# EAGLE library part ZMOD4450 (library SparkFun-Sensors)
ZMOD4450 Food-Ripening Gas Sensor The ZMOD4450 gas sensor module is a software configurable platform designed for detecting gases associated with food ripening or rotting and is targeted for use in refrigeration air quality (RAQ) applications. The sensor is a 12-pin LGA assembly (3.0 x 3.0 x 0.7 mm) that consists of a gas sense element and a CMOS signal conditioning IC. The module’s sense element consists of a micro-heater and sensing material integrated on a silicon-based MEMS structure. It measures the metal oxide (MOx) conductivity, which is a function of the gas concentration. SparkFun Products: SparkFun Refrigeration Gas Sensor ZMOD4450 (Qwiic)
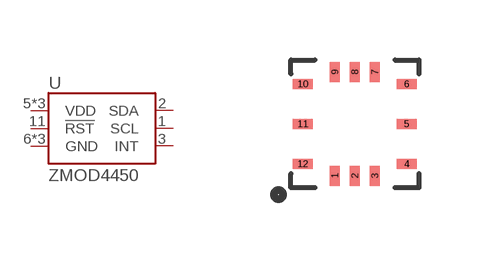
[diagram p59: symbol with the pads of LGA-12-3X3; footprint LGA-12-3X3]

Designator prefix U

## ZMOD4450 (PROD_ID: IC-15106; VALUE: ZMOD4450 Refrigeration Gas Sensor)  [LGA-12-3X3]
1  SCL
2  SDA
3  INT
5  VDD
6  GND
7  GND
9  GND
10  VDD
11  !RST
12  VDD

## Footprint LGA-12-3X3 (pad centres in mm)
12-LGA - 3x3 mm Specifications: Pin count: 12 Pin pitch: 0.50 mm Area: 3x3mm Datasheet referenced for footprint
smd 0.25 x 0.5: 1 -0.5,-1.3; 2 0,-1.3; 3 0.5,-1.3; 7 0.5,1.3; 8 0,1.3; 9 -0.5,1.3
smd 0.5 x 0.25: 4 1.3,-1; 5 1.3,0; 6 1.3,1; 10 -1.3,1; 11 -1.3,0; 12 -1.3,-1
